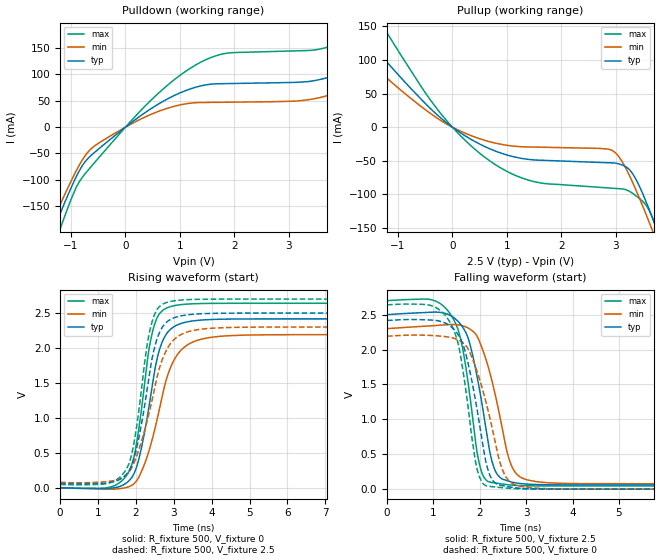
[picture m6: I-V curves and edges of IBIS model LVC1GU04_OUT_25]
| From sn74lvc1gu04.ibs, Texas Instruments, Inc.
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[Model]   LVC1GU04_OUT_25
Model_type  Output
Vref =   0
Rref =   500
Cref =   30p
Vmeas =   1.25
| variable   typ   min   max
C_comp   8.75pF   3.83pF   12.80pF
| C_pullup   9.23pF   5.19pF   12.31pF
| C_pulldown   8.27pF   3.83pF   12.80pF
[Temperature Range]   40   100   -40
| Ambient temperature   25   85   -40
[Voltage range]   2.5   2.3   2.7
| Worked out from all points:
|   slope of the pulldown table from 0 to 0.375 V, typ, clamps not added: 13.1 ohm
|   slope of the pullup table from 0 to 0.375 V, typ, clamps not added: 19.1 ohm
|   rising waveform, R_fixture 500, V_fixture 0: 20-80 % time 490ps typ, 647ps min, 409ps max; typ from 0 V to 2.42 V
|   falling waveform, R_fixture 500, V_fixture 2.5: 20-80 % time 400ps typ, 459ps min, 350ps max; typ from 2.5 V to 0.06 V
|   rising waveform, R_fixture 500, V_fixture 2.5: 20-80 % time 485ps typ, 647ps min, 411ps max; typ from 0.06 V to 2.5 V
|   falling waveform, R_fixture 500, V_fixture 0: 20-80 % time 404ps typ, 505ps min, 354ps max; typ from 2.42 V to 0 V
[Pulldown]
| LVC1GU04_OUT_25
|   Voltage   I(typ)   I(min)   I(max)
-5.5V     -1.282A    -1.18A     -1.449A
-1.445V   -226.9mA   -204.1mA   -265mA
-1.2V     -164.1mA   -147mA     -193mA
-860mV    -85.14mA   -74.3mA    -105.7mA
-470mV    -39.36mA   -28.83mA   -55.6mA
750mV     52.37mA    35.19mA    77.68mA
1.805V    82.52mA    47.23mA    139.3mA
3.895V    100.2mA    65.4mA     158.7mA
4.445V    125.8mA    87.91mA    189.9mA
5.385V    189.1mA    141.7mA    271.5mA
6.1V      249.5mA    192.5mA    350.7mA
11V       818.3mA    670.6mA    1.103A
[Pullup]
| LVC1GU04_OUT_25
|   Voltage   I(typ)   I(min)   I(max)
-5.5V     592.1mA    472.8mA    820.6mA
-2.225V   199.5mA    153.6mA    284.4mA
-1.77V    152.2mA    116.2mA    218.5mA
-1.335V   109.5mA    82.71mA    158.4mA
-185mV    11.75mA    8.511mA    17.46mA
685mV     -32.18mA   -21.72mA   -50.11mA
1.53V     -49.05mA   -29.74mA   -81.74mA
2.935V    -53.28mA   -34.76mA   -90.99mA
3.285V    -66.39mA   -77.56mA   -97.13mA
3.66V     -131.8mA   -150.9mA   -131.8mA
3.745V    -150mA     -168.7mA   -148.9mA
11V       -1.979A    -1.892A    -2.149A
[Ramp]
| LVC1GU04_OUT_25
| variable   typ   min   max
dV/dt_r   1.46/4.98E-10   1.33/6.59E-10   1.59/4.19E-10
dV/dt_f   1.49/4.12E-10   1.37/4.80E-10   1.61/3.64E-10
R_load = 500
[Rising Waveform]
| LVC1GU04_OUT_25
R_fixture =   500
C_fixture =   0
L_fixture =   0
V_fixture =   0
V_fixture_min = 0
V_fixture_max = 0
|   Time   V(typ)   V(min)   V(max)
0s        34.4pV     5.527nV    1.802nV
1.76ns    71.91mV    3.954mV    181.4mV
1.925ns   175mV      46.01mV    387.7mV
2.08ns    416.1mV    154.5mV    856.7mV
2.325ns   1.095V     493.3mV    1.911V
2.49ns    1.657V     818.8mV    2.333V
2.77ns    2.17V      1.485V     2.56V
3.23ns    2.357V     1.989V     2.623V
5.51ns    2.416V     2.189V     2.64V
50ns      2.416V     2.191V     2.64V
[Falling Waveform]
| LVC1GU04_OUT_25
R_fixture =   500
C_fixture =   0
L_fixture =   0
V_fixture =   2.5
V_fixture_min = 2.3
V_fixture_max = 2.7
|   Time   V(typ)   V(min)   V(max)
0s        2.5V       2.3V       2.7V
960ps     2.534V     2.34V      2.712V
1.395ns   2.476V     2.359V     2.477V
1.635ns   2.317V     2.339V     2V
1.91ns    1.72V      2.221V     671.8mV
2.065ns   1.148V     1.991V     201.8mV
2.29ns    339.2mV    1.474V     92.79mV
2.695ns   100.9mV    319mV      57.53mV
4.205ns   60.34mV    78.92mV    45.64mV
50ns      60.06mV    77.04mV    45.59mV
[Rising Waveform]
| LVC1GU04_OUT_25
R_fixture =   500
C_fixture =   0
L_fixture =   0
V_fixture =   2.5
V_fixture_min = 2.3
V_fixture_max = 2.7
|   Time   V(typ)   V(min)   V(max)
0s        60.06mV    77.04mV    45.59mV
1.225ns   65.8mV     86.2mV     57.93mV
1.725ns   176.7mV    170.2mV    245.6mV
1.88ns    309.7mV    275.1mV    463.1mV
2.03ns    594.2mV    468mV      920.6mV
2.295ns   1.401V     956.1mV    2.038V
2.445ns   1.897V     1.298V     2.408V
2.73ns    2.322V     1.881V     2.634V
3.125ns   2.452V     2.171V     2.683V
50ns      2.5V       2.3V       2.7V
[Falling Waveform]
| LVC1GU04_OUT_25
R_fixture =   500
C_fixture =   0
L_fixture =   0
V_fixture =   0
V_fixture_min = 0
V_fixture_max = 0
|   Time   V(typ)   V(min)   V(max)
0s        2.416V     2.191V     2.64V
1.235ns   2.385V     2.186V     2.504V
1.525ns   2.221V     2.14V      2.104V
1.705ns   1.92V      2.05V      1.387V
1.89ns    1.335V     1.783V     469.1mV
2ns       902.6mV    1.563V     163.6mV
2.24ns    164.6mV    953.3mV    37.84mV
2.445ns   56.29mV    361.4mV    23.65mV
2.635ns   32.37mV    115.7mV    11.77mV
50ns      66.72nV    144.1nV    3.207nV
